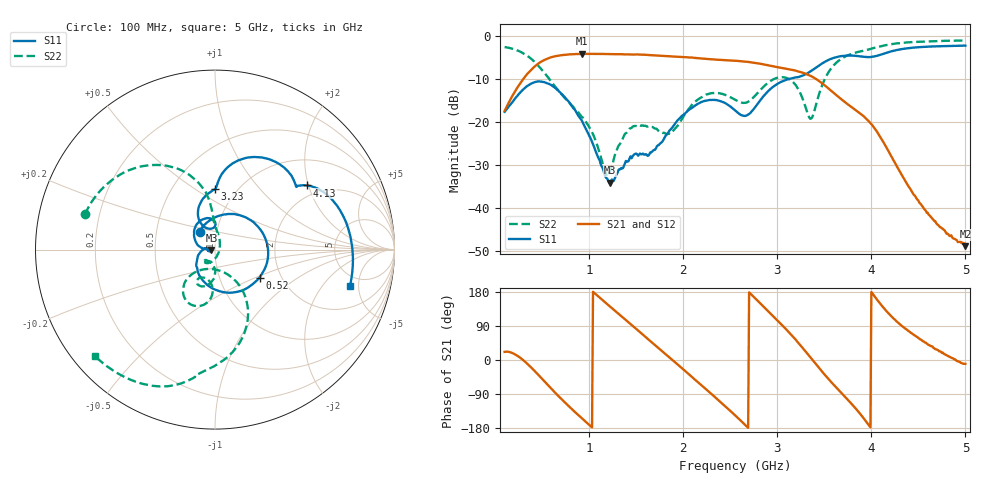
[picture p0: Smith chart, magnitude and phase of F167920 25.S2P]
!  2-Port S-parameters saved by WinCal
! VAR MeasName=S-Parameters (CALIBRATED_DATA) read from VNA (N5242A)
! VAR MeasDate=2016-11-22 9:56:24
! VAR NAME=F167920 25
! VAR FILENAME=F167920 25.S2P
! VAR DATE=2016-11-22 9:56:24
! VAR PHYS_PORTS=1,2
# Hz S DB R 50
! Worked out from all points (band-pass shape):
!   491 points, 100 MHz to 5 GHz, reference 50 ohm
!   highest |S21| = -4.08 dB at 920 MHz (marker M1); lowest = -48.9 dB at 5 GHz (marker M2)
!   |S21| within 3 dB of the highest: 417.2 MHz to 2.976 GHz (2.559 GHz wide, 151 % of centre)
!   lowest |S11| = -34.1 dB at 1.22 GHz (marker M3), VSWR 1.04, Z = 48.1 - j0.165 ohm
!   |S11| at or under -10 dB: start of sweep to 3.115 GHz
!   |S22| runs from -32.6 to -1.0 dB; largest |S21 - S12| = 0.0012
!   S11 on the Smith chart (normalised r, x): 100 MHz: 0.83, +0.17; 520 MHz: 1.55, -0.53; 3.23 GHz: 0.80, +0.61; 4.13 GHz: 1.67, +1.97; 5 GHz: 3.87, -3.95
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1e8  -17.58 130.5  -17.38 21.4  -17.38 21.4  -2.50 164.8
3e8  -12.33 50.1  -9.89 -0.9  -9.89 -0.9  -3.98 133.9
5.2e8  -10.66 -32.2  -5.54 -55.6  -5.54 -55.5  -8.42 103.6
7e8  -13.25 -93.3  -4.41 -102.0  -4.41 -102.0  -13.36 94.3
9.2e8  -19.57 -157.2  -4.08 -153.4  -4.07 -153.4  -18.75 87.5
1.18e9  -32.98 173.0  -4.13 149.9  -4.13 149.9  -32.14 0.3
1.22e9  -34.08 -175.0  -4.14 141.3  -4.15 141.3  -31.49 -43.3
1.44e9  -27.95 -173.6  -4.22 94.9  -4.22 94.9  -21.42 -120.0
1.74e9  -25.32 173.7  -4.48 30.7  -4.49 30.7  -22.09 -132.4
1.96e9  -19.12 160.2  -4.79 -16.2  -4.79 -16.2  -20.12 -92.8
2.19e9  -15.32 128.1  -5.17 -66.0  -5.19 -66.0  -14.24 -99.7
2.37e9  -14.93 101.7  -5.46 -105.1  -5.47 -105.1  -13.22 -114.8
2.55e9  -17.22 88.9  -5.69 -145.7  -5.70 -145.7  -14.75 -119.3
2.73e9  -17.44 113.5  -6.08 171.3  -6.08 171.2  -14.57 -97.5
2.93e9  -12.20 112.3  -6.87 122.1  -6.88 122.1  -10.37 -99.3
3.23e9  -9.45 89.7  -8.23 43.3  -8.23 43.3  -12.59 -133.3
3.37e9  -7.91 86.2  -9.39 1.4  -9.41 1.4  -18.87 -84.0
3.62e9  -4.90 64.7  -13.56 -70.9  -13.59 -70.8  -6.30 -69.8
4.13e9  -4.06 34.8  -24.72 137.7  -24.76 138.0  -2.17 -105.4
4.19e9  -3.64 31.6  -27.05 121.0  -27.08 121.5  -1.91 -108.7
4.57e9  -2.44 7.3  -40.36 46.1  -40.51 48.6  -1.20 -125.6
5e9  -2.17 -14.9  -48.85 -10.1  -48.35 -12.4  -0.97 -138.5
